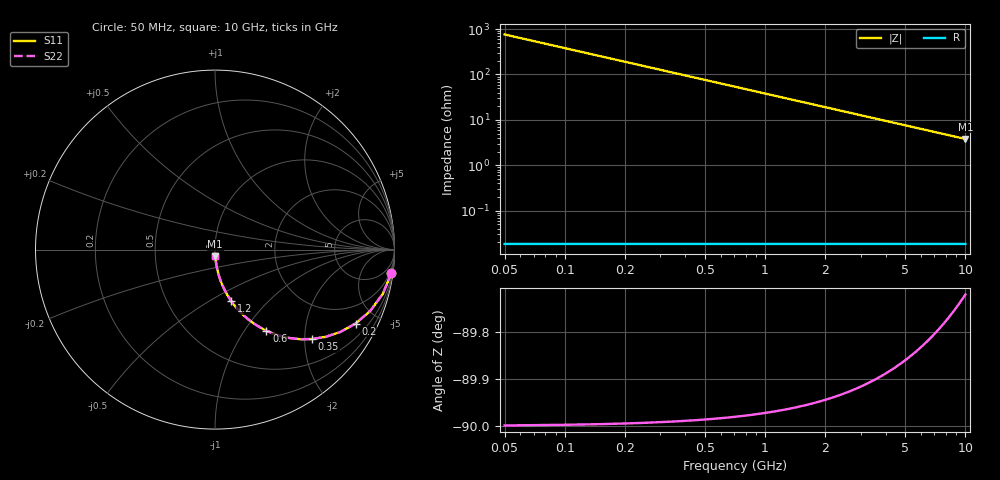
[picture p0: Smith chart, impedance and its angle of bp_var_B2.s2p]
! Created Fri Sep 21 13:01:53 2018
# ghz S ma R 50
! 2 Port Network Data from SP1.SP block
! freq  magS11  angS11  magS21  angS21  magS12  angS12  magS22  angS22
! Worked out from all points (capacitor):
!   200 points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, 50 MHz to 10 GHz, reference 50 ohm
!   read as one part in series: C = 4.19 pF near 100 MHz
!   lowest |Z| = 3.8 ohm at 10 GHz (marker M1)
!   S11 on the Smith chart (normalised r, x): 50 MHz: 1, -15; 200 MHz: 1.00, -3.80; 350 MHz: 1.00, -2.17; 600 MHz: 1.00, -1.27; 1.2 GHz: 1.00, -0.63; 10 GHz: 1.00, -0.08
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0.05  0.9915 -7.5  0.1304 82.5  0.1304 82.5  0.9915 -7.5
0.1  0.9671 -14.7  0.2544 75.3  0.2544 75.3  0.9671 -14.7
0.15  0.9302 -21.5  0.3671 68.5  0.3671 68.5  0.9302 -21.5
0.2  0.8849 -27.8  0.4656 62.2  0.4656 62.2  0.8849 -27.8
0.25  0.8354 -33.3  0.5495 56.7  0.5495 56.7  0.8354 -33.3
0.3  0.7849 -38.3  0.6195 51.7  0.6195 51.7  0.7849 -38.3
0.35  0.7356 -42.6  0.6773 47.4  0.6773 47.4  0.7356 -42.6
0.45  0.6452 -49.8  0.7639 40.2  0.7639 40.2  0.6452 -49.8
0.5  0.6051 -52.7  0.796 37.2  0.796 37.2  0.6051 -52.7
0.6  0.5351 -57.6  0.8446 32.3  0.8446 32.3  0.5351 -57.6
0.7  0.4771 -61.5  0.8787 28.5  0.8787 28.5  0.4771 -61.5
0.85  0.4082 -65.9  0.9127 24.1  0.9127 24.1  0.4082 -65.9
1  0.3552 -69.2  0.9346 20.8  0.9346 20.8  0.3552 -69.2
1.2  0.3019 -72.4  0.9532 17.6  0.9532 17.6  0.3019 -72.4
1.75  0.2122 -77.7  0.977 12.3  0.977 12.3  0.2122 -77.7
2.5  0.1503 -81.3  0.9885 8.6  0.9885 8.6  0.1503 -81.3
3.4  0.1111 -83.5  0.9936 6.4  0.9936 6.4  0.1111 -83.5
4.15  0.09119 -84.7  0.9956 5.2  0.9956 5.2  0.09119 -84.7
5.05  0.07504 -85.6  0.997 4.3  0.997 4.3  0.07504 -85.6
6.7  0.05663 -86.6  0.9982 3.2  0.9982 3.2  0.05663 -86.6
8.35  0.04547 -87.2  0.9988 2.6  0.9988 2.6  0.04547 -87.2
10  0.03798 -87.5  0.9991 2.2  0.9991 2.2  0.03798 -87.5
